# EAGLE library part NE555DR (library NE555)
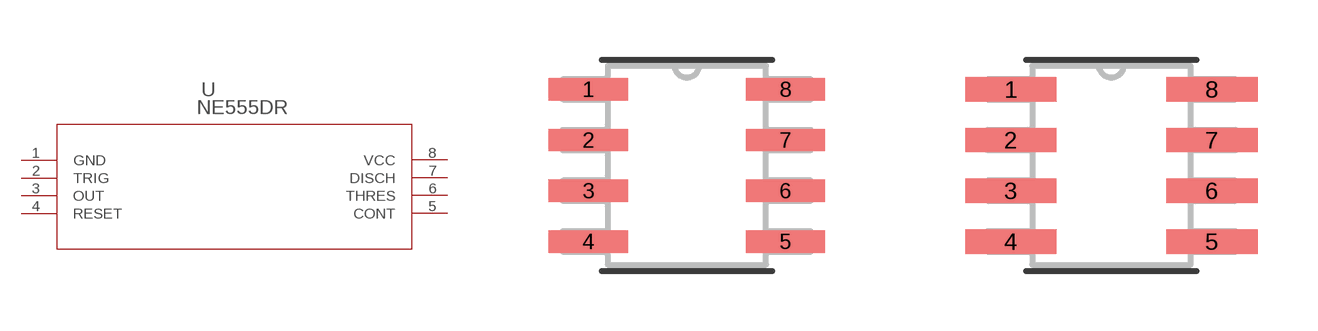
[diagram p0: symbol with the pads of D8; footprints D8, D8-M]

Designator prefix U

## NE555DR (MANUFACTURER_PART_NUMBER: NE555DR; VENDOR: Vendor)  [D8]
1  GND  pwr
2  TRIG  in
3  OUT  out
4  RESET  in
5  CONT  pas
6  THRES  in
7  DISCH  pas
8  VCC  pwr

## NE555DRD8-M (MANUFACTURER_PART_NUMBER: NE555DR; VENDOR: Vendor)  [D8-M]
Pads as for D8

## NE555DRD8-L (MANUFACTURER_PART_NUMBER: NE555DR; VENDOR: Vendor)  [D8-L]
Pads as for D8

## Footprint D8 (pad centres in mm)
smd 1.981 x 0.559: 1 -2.464,1.905; 2 -2.464,0.635; 3 -2.464,-0.635; 4 -2.464,-1.905; 5 2.464,-1.905; 6 2.464,-0.635; 7 2.464,0.635; 8 2.464,1.905

## Footprint D8-M (pad centres in mm)
smd 2.286 x 0.61: 1 -2.515,1.905; 2 -2.515,0.635; 3 -2.515,-0.635; 4 -2.515,-1.905; 5 2.515,-1.905; 6 2.515,-0.635; 7 2.515,0.635; 8 2.515,1.905

## Footprint D8-L (pad centres in mm)
smd 1.676 x 0.508: 1 -2.413,1.905; 2 -2.413,0.635; 3 -2.413,-0.635; 4 -2.413,-1.905; 5 2.413,-1.905; 6 2.413,-0.635; 7 2.413,0.635; 8 2.413,1.905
